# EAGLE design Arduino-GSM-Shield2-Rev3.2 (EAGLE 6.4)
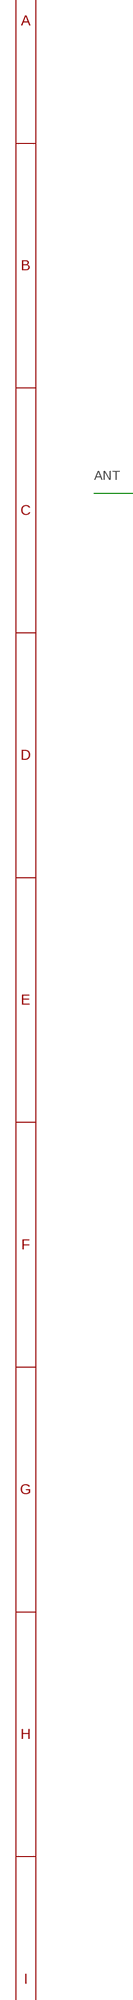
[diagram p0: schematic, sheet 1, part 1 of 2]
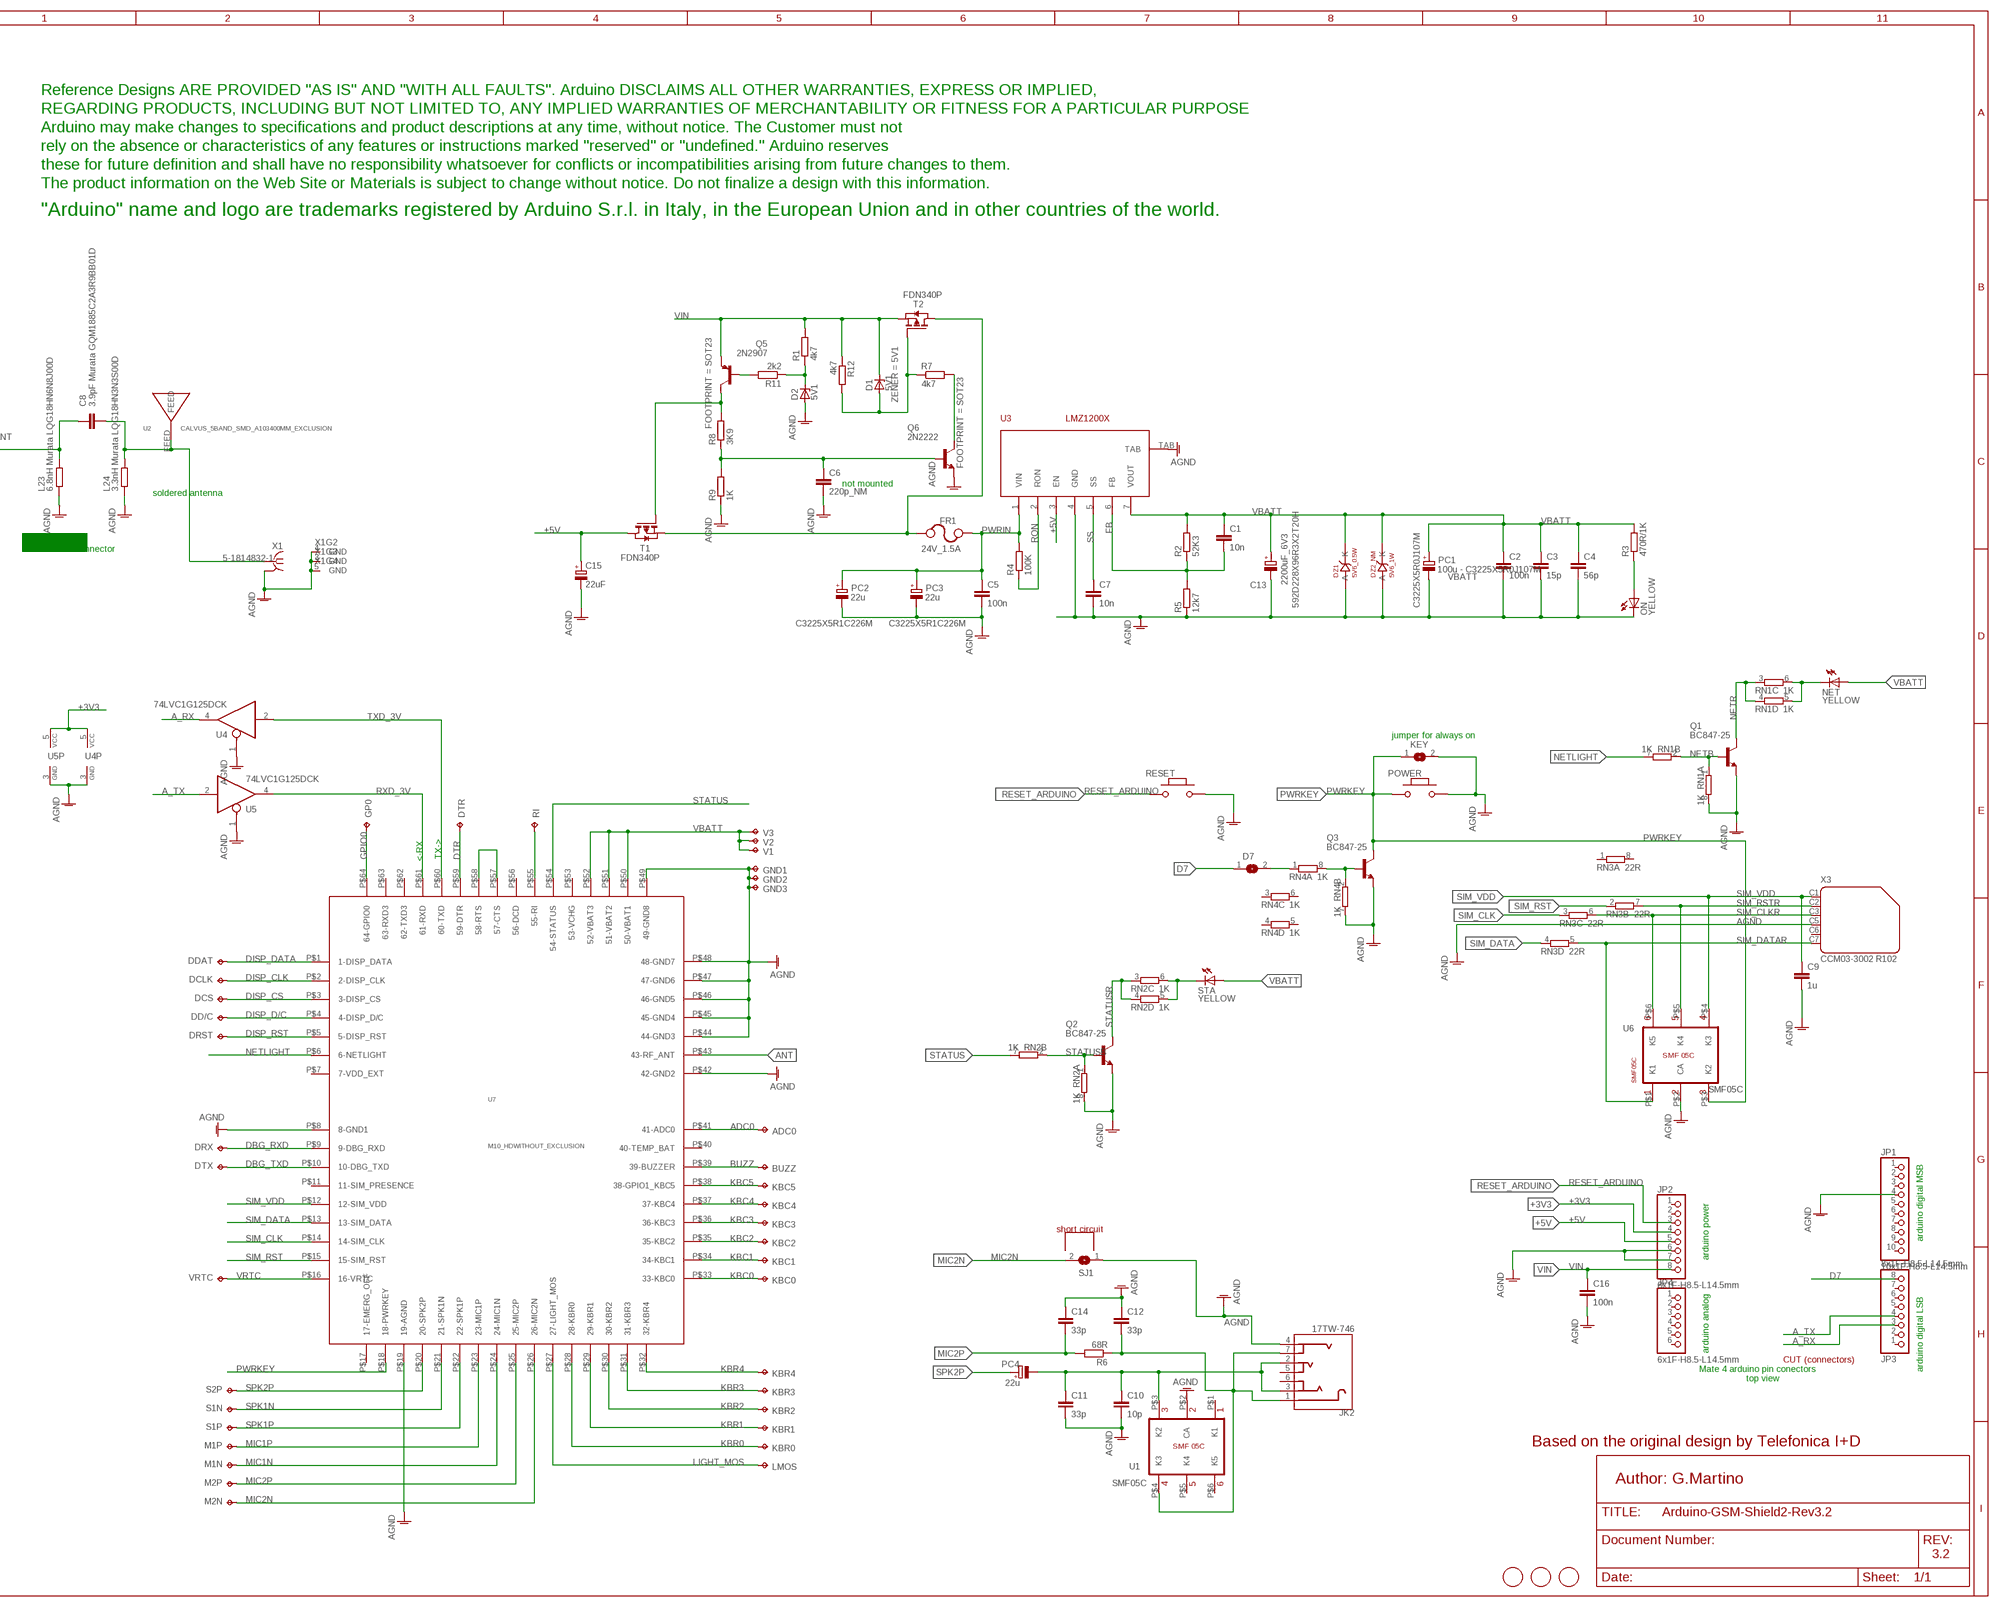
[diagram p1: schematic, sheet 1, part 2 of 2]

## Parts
ADC0  TPPAD1-09  [P1-09]
BUZZ  TPPAD1-09  [P1-09]
C1  10n  C-EU0603-RND  [C0603-ROUND]
C2  100n  C-EU0603-RND  [C0603-ROUND]
C3  15p  C-EU0603-RND  [C0603-ROUND]
C4  56p  C-EU0603-RND  [C0603-ROUND]
C5  100n  C-EU0603-RND  [C0603-ROUND]
C6  220p_NM  C-EU0603-RND  [C0603-ROUND]
C7  10n  C-EU0603-RND  [C0603-ROUND]
C8  3.9pF Murata GQM1885C2A3R9BB01D  C-EU0603-RND  [C0603-ROUND]
C9  1u  C-EU0603-RND  [C0603-ROUND]
C10  10p  C-EU0603-RND  [C0603-ROUND]
C11  33p  C-EU0603-RND  [C0603-ROUND]
C12  33p  C-EU0603-RND  [C0603-ROUND]
C13  2200uF_6V3  0348_  [592D-X]
C14  33p  C-EU0603-RND  [C0603-ROUND]
C15  22uF  0167_  [SMC_B]
C16  100n  C-EU0603-RND  [C0603-ROUND]
D1  5V1  ZENER-DIODESMB  [SMB]
D2  5V1  ZENER-DIODESMB  [SMB]
D7  SJ  [SJ]
DCLK  TPPAD1-09  [P1-09]
DCS  TPPAD1-09  [P1-09]
DD/C  TPPAD1-09  [P1-09]
DDAT  TPPAD1-09  [P1-09]
DRST  TPPAD1-09  [P1-09]
DRX  TPPAD1-09  [P1-09]
DTR  TPPAD1-09  [P1-09]
DTX  TPPAD1-09  [P1-09]
DZ1  5V6_0.5W  0433_BZM55B5V6-TR  [MICROMELF-R]
DZ2_NM  5V6_1W  0433_BZM55B5V6-TR_MINIMELF  [MINIMELF]
FR1  24V_1.5A  0319_MF-MSMF150/24X-2_(24V)  [MF-MSMF-S2]
GND1  TPPAD1-09  [P1-09]
GND2  TPPAD1-09  [P1-09]
GND3  TPPAD1-09  [P1-09]
GP0  TPPAD1-09  [P1-09]
JK2  17TW-746  1819_17TW-746  [17TW-746]
JP1  10x1F-H8.5-L14.5mm  PINHD-1X10TH  [1X10-TH]
JP2  8x1F-H8.5-L14.5mm  PINHD-1X8TH  [1X08-TH]
JP3  8x1F-H8.5-L14.5mm  PINHD-1X8TH  [1X08-TH]
JP4  6x1F-H8.5-L14.5mm  PINHD-1X6TH  [1X06-TH]
KBC0  TPPAD1-09  [P1-09]
KBC1  TPPAD1-09  [P1-09]
KBC2  TPPAD1-09  [P1-09]
KBC3  TPPAD1-09  [P1-09]
KBC4  TPPAD1-09  [P1-09]
KBC5  TPPAD1-09  [P1-09]
KBR0  TPPAD1-09  [P1-09]
KBR1  TPPAD1-09  [P1-09]
KBR2  TPPAD1-09  [P1-09]
KBR3  TPPAD1-09  [P1-09]
KBR4  TPPAD1-09  [P1-09]
KEY  SJ  [SJ]
L23  6.8nH Murata LQG18HN6N8J00D  R-EU_0603-RND  [R0603-ROUND]
L24  3.3nH Murata LQG18HN3N3S00D  R-EU_0603-RND  [R0603-ROUND]
LMOS  TPPAD1-09  [P1-09]
M1N  TPPAD1-09  [P1-09]
M1P  TPPAD1-09  [P1-09]
M2N  TPPAD1-09  [P1-09]
M2P  TPPAD1-09  [P1-09]
NET  YELLOW  LEDCHIP-LED0805  [CHIP-LED0805]
ON  YELLOW  LEDCHIP-LED0805  [CHIP-LED0805]
PC1  100u - C3225X5R0J107M  CPOL-EUSMCB  [SMC_B]
PC2  22u  CPOL-EUSMCB  [SMC_B]
PC3  22u  CPOL-EUSMCB  [SMC_B]
PC4  22u  CPOL-EUSMCB  [SMC_B]
POWER  MYSMD_PB157  [SMD_157SW]
Q1  BC847-25  BC817-25SMD  [SOT23-BEC]
Q2  BC847-25  BC817-25SMD  [SOT23-BEC]
Q3  BC847-25  BC817-25SMD  [SOT23-BEC]
Q5  2N2907  MMBT2907ALT1-PNP-SOT23-BEC  [SOT23-BEC]
Q6  2N2222  MMBT2222ALT1-NPN-SOT23-BEC  [SOT23-BEC]
R1  4k7  R-EU_0603-RND  [R0603-ROUND]
R2  52K3  R-EU_0603-RND  [R0603-ROUND]
R3  470R/1K  R-EU_0603-RND  [R0603-ROUND]
R4  100K  R-EU_0603-RND  [R0603-ROUND]
R5  12k7  R-EU_0603-RND  [R0603-ROUND]
R6  68R  R-EU_0603-RND  [R0603-ROUND]
R7  4k7  R-EU_0603-RND  [R0603-ROUND]
R8  3K9  R-EU_0603-RND  [R0603-ROUND]
R9  1K  R-EU_0603-RND  [R0603-ROUND]
R11  2k2  R-EU_0603-RND  [R0603-ROUND]
R12  4k7  R-EU_0603-RND  [R0603-ROUND]
RESET  MYSMD_PB157  [SMD_157SW]
RI  TPPAD1-09  [P1-09]
RN1  1K  4R-NCAY16  [CAY16]
RN2  1K  4R-NCAY16  [CAY16]
RN3  22R  4R-NCAY16  [CAY16]
RN4  1K  4R-NCAY16  [CAY16]
S1N  TPPAD1-09  [P1-09]
S1P  TPPAD1-09  [P1-09]
S2P  TPPAD1-09  [P1-09]
SJ1  SJ  [SJ]
STA  YELLOW  LEDCHIP-LED0805  [CHIP-LED0805]
T1  FDN340P  PMOSSOT23  [SOT-23]
T2  FDN340P  PMOSSOT23  [SOT-23]
U1  SMF05C  [SC70_6L]
U2  CALVUS_5BAND_SMD_A103400MM_EXCLUSION  [CALVUS_5BAND_SMD_A10340_0MM_EXCLUSION]
U3  LMZ1200X  [TZA-7]
U4  74LVC1G125DCK  [SC70-5]
U5  74LVC1G125DCK  [SC70-5]
U6  SMF05C  [SC70_6L]
U7  M10_HDWITHOUT_EXCLUSION  [M10_HD_WITHOUT_EXCLUSION]
U$1  FIDUCIALMOUNT  [FIDUCIA-MOUNT]
U$2  FIDUCIALMOUNT  [FIDUCIA-MOUNT]
U$3  FIDUCIALMOUNT  [FIDUCIA-MOUNT]
U$4  DISCLAIMER  [DISCLAIMER]
V1  TPPAD1-09  [P1-09]
V2  TPPAD1-09  [P1-09]
V3  TPPAD1-09  [P1-09]
VRTC  TPPAD1-09  [P1-09]
X1  0633_5-1814832-1  [BU-SMA-V]
X3  CCM03-3002 R102  0575_CCM03-3002_R102  [CON-AMPHENOL_C707_10M006_512_2]

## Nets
+3V3: JP2.4 U4.5(VCC) U5.5(VCC)
+5V: C15.+ JP2.5 T1.1(D) U3.3(EN)
A_RX: JP3.3 U4.4(O)
A_TX: JP3.4 U5.2(I)
ADC0: ADC0.TP U7.P$41(41-ADC0)
AGND: C2.2 C3.2 C4.2 C5.2 C6.2 C7.2 C9.2 C10.2 C11.2 C12.1 C13.- C14.1 C15.- C16.2 D2.A DZ1.A DZ2_NM.A GND1.TP GND2.TP GND3.TP JK2.4 JP1.4 JP2.6 JP2.7 KEY.2 L23.1 L24.1 ON.C PC1.- PC2.- PC3.- POWER.2 Q1.E Q2.E Q3.E Q6.E R5.1 R9.1 RESET.2 RN1.8 RN2.8 RN4.7 SJ1.1 U1.P$2(CA) U3.4(GND) U3.TAB U4.1(OE) U4.3(GND) U5.1(OE) U5.3(GND) U6.P$2(CA) U7.P$8(8-GND1) U7.P$19(19-AGND) U7.P$42(42-GND2) U7.P$44(44-GND3) U7.P$45(45-GND4) U7.P$46(46-GND5) U7.P$47(47-GND6) U7.P$48(48-GND7) U7.P$49(49-GND8) X1.2(GND) X1.3(GND) X1.4(GND) X1.5(GND) X3.C5
ANT [antenna]: C8.1 L23.2 U7.P$43(43-RF_ANT)
ANTENA [antenna]: C8.2 L24.2 U2.FEED X1.1
BUZZ: BUZZ.TP U7.P$39(39-BUZZER)
D7: D7.1 JP3.8
DBG_RXD: DRX.TP U7.P$9(9-DBG_RXD)
DBG_TXD: DTX.TP U7.P$10(10-DBG_TXD)
DISP_CLK: DCLK.TP U7.P$2(2-DISP_CLK)
DISP_CS: DCS.TP U7.P$3(3-DISP_CS)
DISP_D/C: DD/C.TP U7.P$4(4-DISP_D/C)
DISP_DATA: DDAT.TP U7.P$1(1-DISP_DATA)
DISP_RST: DRST.TP U7.P$5(5-DISP_RST)
DTR: DTR.TP U7.P$59(59-DTR)
FB: C1.2 R2.1 R5.2 U3.6(FB)
GPIO0: GP0.TP U7.P$64(64-GPIO0)
KBC0: KBC0.TP U7.P$33(33-KBC0)
KBC1: KBC1.TP U7.P$34(34-KBC1)
KBC2: KBC2.TP U7.P$35(35-KBC2)
KBC3: KBC3.TP U7.P$36(36-KBC3)
KBC4: KBC4.TP U7.P$37(37-KBC4)
KBC5: KBC5.TP U7.P$38(38-GPIO1_KBC5)
KBR0: KBR0.TP U7.P$28(28-KBR0)
KBR1: KBR1.TP U7.P$29(29-KBR1)
KBR2: KBR2.TP U7.P$30(30-KBR2)
KBR3: KBR3.TP U7.P$31(31-KBR3)
KBR4: KBR4.TP U7.P$32(32-KBR4)
LIGHT_MOS: LMOS.TP U7.P$27(27-LIGHT_MOS)
MIC1N: M1N.TP U7.P$24(24-MIC1N)
MIC1P: M1P.TP U7.P$23(23-MIC1P)
MIC2N: M2N.TP SJ1.2 U7.P$26(26-MIC2N)
MIC2P: C14.2 M2P.TP R6.2 U7.P$25(25-MIC2P)
N$1: U7.P$57(57-CTS) U7.P$58(58-RTS)
N$2: RI.TP U7.P$55(55-RI)
N$3: ON.A R3.1
N$4: Q3.B RN4.2 RN4.8
N$6: C12.2 JK2.1 JK2.7 R6.1 U1.P$4(K3)
N$7: D7.2 RN4.1
N$8: Q6.C R7.2
N$9: Q5.C R8.2 T1.3(G)
N$10: Q5.B R11.2
N$11: C6.1 Q6.B R8.1 R9.2
N$12: C10.1 C11.1 JK2.2 JK2.3 PC4.- U1.P$3(K2)
N$13: D1.A R7.1 R12.2 T2.3(G)
N$14: D2.C R1.1 R11.1
N$15: FR1.P$1 T1.2(S) T2.1(D)
NETB: Q1.B RN1.1 RN1.2
NETL: NET.C RN1.5 RN1.6
NETLIGHT: RN1.7 U7.P$6(6-NETLIGHT)
NETR: Q1.C RN1.3 RN1.4
PWRIN: C5.1 FR1.P$2 PC2.+ PC3.+ R4.2 U3.1(VIN)
PWRKEY: KEY.1 POWER.1 Q3.C U6.P$3(K2) U7.P$18(18-PWRKEY)
RESET_ARDUINO: JP2.3 RESET.1
RON: R4.1 U3.2(RON)
RXD_3V: U5.4(O) U7.P$61(61-RXD)
SIM_CLK: RN3.3 U7.P$14(14-SIM_CLK)
SIM_CLKR: RN3.6 U6.P$6(K5) X3.C3
SIM_DATA: RN3.4 U7.P$13(13-SIM_DATA)
SIM_DATAR: RN3.5 U6.P$1(K1) X3.C7
SIM_RST: RN3.2 U7.P$15(15-SIM_RST)
SIM_RSTR: RN3.7 U6.P$5(K4) X3.C2
SIM_VDD: C9.1 U6.P$4(K3) U7.P$12(12-SIM_VDD) X3.C1
SPK1N: S1N.TP U7.P$21(21-SPK1N)
SPK1P: S1P.TP U7.P$22(22-SPK1P)
SPK2P: PC4.+ S2P.TP U7.P$20(20-SPK2P)
SS: C7.1 U3.5(SS)
STATUS: RN2.7 U7.P$54(54-STATUS)
STATUSB: Q2.B RN2.1 RN2.2
STATUSL: RN2.5 RN2.6 STA.C
STATUSR: Q2.C RN2.3 RN2.4
TXD_3V: U4.2(I) U7.P$60(60-TXD)
VBATT: C1.1 C2.1 C3.1 C4.1 C13.+ DZ1.C(K) DZ2_NM.C(K) NET.A PC1.+ R2.2 R3.2 STA.A U3.7(VOUT) U7.P$50(50-VBAT1) U7.P$51(51-VBAT2) U7.P$52(52-VBAT3) V1.TP V2.TP V3.TP
VIN: C16.1 D1.C JP2.8 Q5.E R1.2 R12.1 T2.2(S)
VRTC: U7.P$16(16-VRTC) VRTC.TP
Unconnected: JK2.5 JK2.6 JP1.1 JP1.2 JP1.3 JP1.5 JP1.6 JP1.7 JP1.8 JP1.9 JP1.10 JP2.1 JP2.2 JP3.1 JP3.2 JP3.5 JP3.6 JP3.7 JP4.1 JP4.2 JP4.3 JP4.4 JP4.5 JP4.6 RN3.1 RN3.8 RN4.3 RN4.4 RN4.5 RN4.6 U1.P$1(K1) U1.P$5(K4) U1.P$6(K5) U7.P$7(7-VDD_EXT) U7.P$11(11-SIM_PRESENCE) U7.P$17(17-EMERG_OFF) U7.P$40(40-TEMP_BAT) U7.P$53(53-VCHG) U7.P$56(56-DCD) U7.P$62(62-TXD3) U7.P$63(63-RXD3) X3.C6

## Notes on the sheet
- not mounted
- soldered antenna
- SMA or U.FL connector
- 592D228X96R3X2T20H
- jumper for always on
- <-RX
- TX->
- SMF05C
- short circuit
- arduino digital MSB
- arduino power
- arduino analog
- CUT (connectors)
- Mate 4 arduino pin conectors | arduino digital LSB
- top view
- Based on the original design by Telefonica I+D
- Author: G.Martino
- 3.2

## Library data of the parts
ADC0 BUZZ DCLK DCS DD/C DDAT DRST DRX DTR DTX GND1-GND3 GP0 KBC0 KBC1-KBC5 KBR0 KBR1-KBR4 LMOS M1N M1P M2N M2P RI S1N S1P S2P V1-V3 VRTC = testpad:TP: Test pad
C1-C12 C14 C16 = SmartPrj:C-EU: CAPACITOR, European symbol
C13 = Condensatori:0348_: 2200uF 16V Elettr. V � Tantalio; MONTHLY_USAGE: 546.27; TYPE: Condensatori
C15 = Condensatori:0167_: 22uF 25V; MONTHLY_USAGE: 319.15; PRICE: �_0.12; SUPPLIER: La_Tecnika_Due_s.r.l.; TYPE: Condensatori
D1 = diode:ZENER-DIODE: Z-Diode; ZENER: 5V1
D2 = diode:ZENER-DIODE: Z-Diode
D7 KEY = jumper:SJ: SMD solder JUMPER
DZ1 = Diodi:0433_BZM55B5V6-TR: Small Signal Zener Diode BZM55B5V6-TR; CASE: MicroMELF/SOD323/SOD110; MONTHLY_USAGE: 0; PART_NUMBER: BZM55B5V6-TR; SUPPLIER: La_Tecnika_Due_s.r.l.; TYPE: Diodi
DZ2_NM = Diodi:0433_BZM55B5V6-TR: Small Signal Zener Diode BZM55B5V6-TR
FR1 = Protezione:0319_MF-MSMF150/24X-2_(24V): MF-MSMF150/24X-2 (24V) -Polyfuse; MONTHLY_USAGE: 0; PART_NUMBER: MF-MSMF150/24X-2_(24V); PRICE: �_0.11; SUPPLIER: La_Tecnika_Due_s.r.l.; TYPE: Protezione
JK2 = Connettori:1819_17TW-746: Audio Jack 3,5mm for mobiles SMD
JP1 = SmartPrj:PINHD-1X10: PIN HEADER
JP2 JP3 = SmartPrj:PINHD-1X8: PIN HEADER
JP4 = SmartPrj:PINHD-1X6: PIN HEADER
L23 L24 R1-R9 R11 R12 = SmartPrj:R-EU_: RESISTOR, European symbol
NET ON STA = led:LED: LED
PC1 = rcl:CPOL-EU: POLARIZED CAPACITOR, European symbol; PN: C3225X5R0J107M
PC2-PC4 = rcl:CPOL-EU: POLARIZED CAPACITOR, European symbol; PN: C3225X5R1C226M
POWER RESET = SmartPrj:MYSMD_PB157
Q1-Q3 = transistor-npn:BC817*: NPN Transistor
Q5 = transistor-neu-to92:*-PNP-: PNP Transistror; FOOTPRINT: SOT23
Q6 = transistor-neu-to92:*-NPN-: NPN Transistror; FOOTPRINT: SOT23
RN1-RN4 = resistor-dil:4R-N: Array Chip Resistor Source: RS Component / Phycomp
SJ1 = SmartPrj:SJ: SMD solder JUMPER
T1 T2 = zetex:PMOSSOT23: MOS FET
U1 U6 = SmartPrj:SMF05C: SMF05C-TVS Diode Array For ESD and Latch-Up Protection
U2 = SmartPrj:CALVUS_5BAND_SMD_A10340
U3 = SmartPrj:LMZ1200X
U4 U5 = 74xx-little-us:74*1G125: Single Bus Buffer Gate with 3-State Output
U7 = GSM:M10_HD
U$1-U$3 = SmartPrj:FIDUCIALMOUNT
U$4 = Misc:DISCLAIMER
X1 = Connettori:0633_5-1814832-1: SMA STRAIGHT PCB SOCKET DIE CAST; MONTHLY_USAGE: _____; PN: 5-1814832-1; PRICE: _____; SUPPLIER: _____; TYPE: Connettori; VALUE: 5-1814832-1
X3 = Connettori:0575_CCM03-3002_R102: CCM03-3002 R102; MONTHLY_USAGE: _____; PART_NUMBER: CCM03-3002_R102; PRICE: _____; SUPPLIER: _____; TYPE: Connettori

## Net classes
1 power: width 0.305 mm, drill 0.406 mm, clearance 0.178 mm
2 gnd: width 0.305 mm, drill 0.406 mm, clearance 0.178 mm
3 power usb: width 0.508 mm, drill 0.406 mm, clearance 0.178 mm
4 antenna: clearance 0.61 mm

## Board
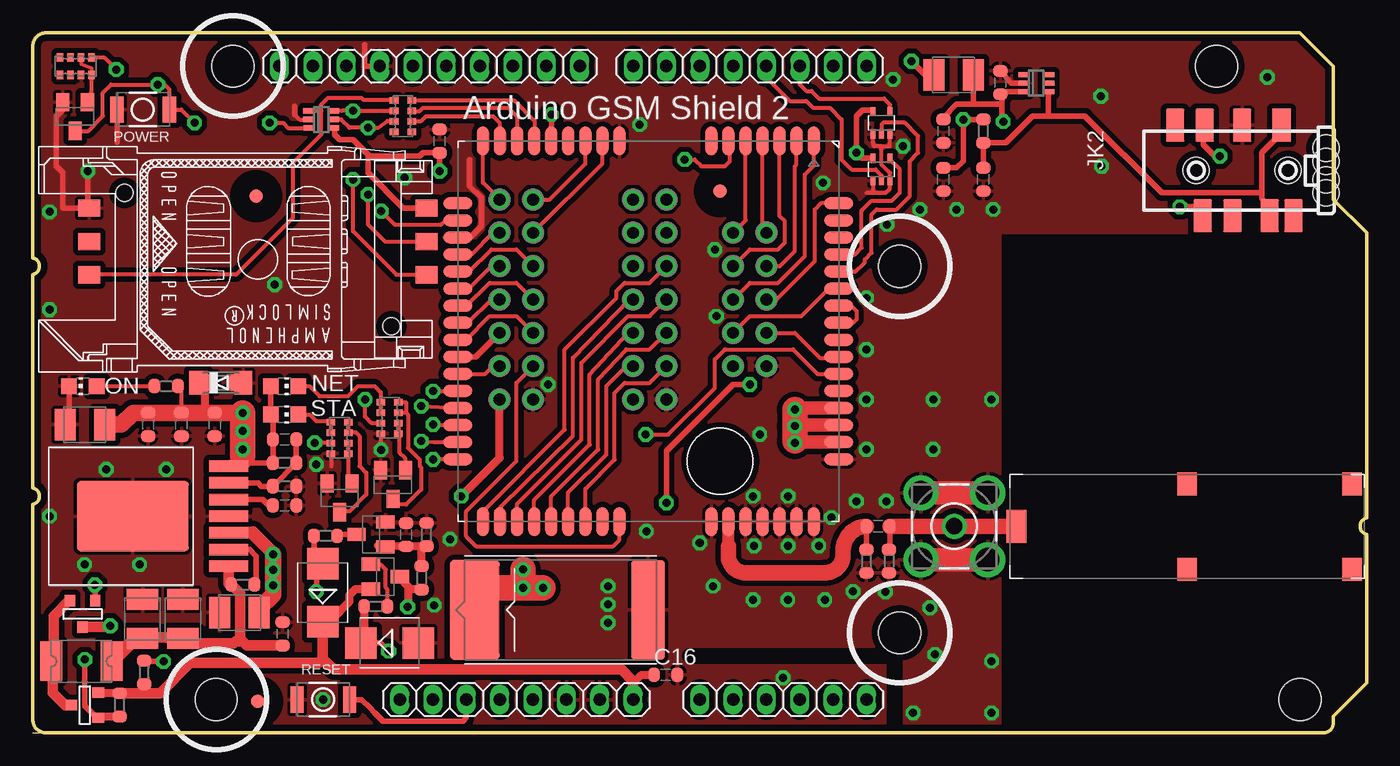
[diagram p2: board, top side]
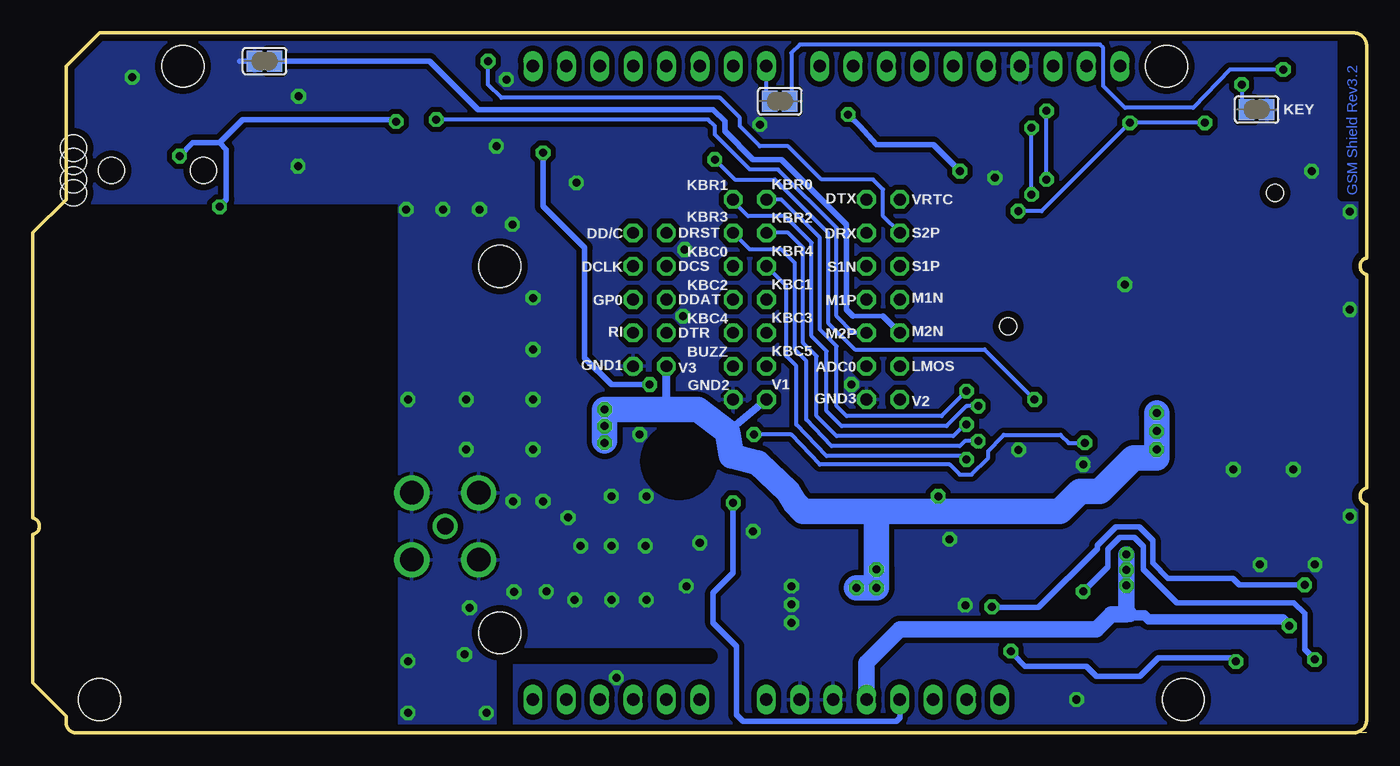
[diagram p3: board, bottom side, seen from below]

Size 101.6 x 53.34 mm. Coordinates in mm from the lower left corner, seen from the top.
Outline: 0,0 77.09,0
Outline: 77.09,0 1,0 arc-90 0,1 0,17.4 arc155 0,18.67 0,34.92 arc155 0,36.2 0,52.34 arc-90 1,53.34 96.52,53.34 99.06,50.8 99.06,40.64 101.6,38.1 101.6,16.38 arc155 101.6,15.11 101.6,3.81 99.06,1.27 99.06,0.76 arc-90 98.3,0 77.09,0
Copper layers (1*16): Top 0.035mm / dielectric 1.5mm / Bottom 0.035mm
Design rules "default *": minimum track width 10mil, minimum drill 24mil, track to track 8mil, track to pad 8mil, pad to pad 8mil, via to via 10mil, smd to smd 8mil, copper to edge 20mil, drill to drill 12mil, minimum pad ring 10mil, minimum via ring 10mil, stop-mask expansion 1mil, vias tented up to drill 30mil, thermal gap 10mil
Holes 3.2 mm at 66.04,35.56 66.04,7.62 15.24,50.8 13.97,2.54 96.52,2.54 90.17,50.8
tRestrict: area 74.9,16.6 to 76.8,18.4; 4 lines
bRestrict: area 0.3,40.9 to 1.8,52.8; 2 lines

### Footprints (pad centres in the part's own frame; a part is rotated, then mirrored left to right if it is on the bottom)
P1-09 = drill 0.9 pad 1.422 octagon: TP 0,0
C0603-ROUND = smd 0.898 x 1.1: 1 -0.889,0; 2 0.889,0
592D-X = smd 7.62 x 3.81: + 0,5.588 | smd 7.62 x 2.54: - 0,-7.62
SMC_B = smd 1.6 x 2.4: + -1.5,0; - 1.5,0
SMB = smd 2.4 x 2.4: A 2.2,0; C -2.2,0
SJ = smd 1.168 x 1.6: 1 -0.762,0; 2 0.762,0
MICROMELF-R = smd 0.8 x 1.2: A 0.8,0; C -0.8,0
MINIMELF = smd 1.4 x 1.8: A 1.7,0; C -1.7,0
MF-MSMF-S2 = smd 1.7 x 3: P$1 -2.3,0; P$2 2.3,0
17TW-746 = smd 1.4 x 2.5: 1 2.8,-3.45; 2 8.8,3.45; 3 8.65,-3.45; 4 5.8,-3.45; 5 10.9,-3.45; 6 6.55,3.45; 7 3.7,3.45; 8 1.9,3.45 | hole 2: 9.3,0; -0.6,1.7; -0.6,-1.7; -0.6,0.7; -0.6,-0.7; 2.3,0
1X10-TH = drill 0.95 pad 1.422 long: 1 -11.43,0; 2 -8.89,0; 3 -6.35,0; 4 -3.81,0; 5 -1.27,0; 6 1.27,0; 7 3.81,0; 8 6.35,0; 9 8.89,0; 10 11.43,0
1X08-TH = drill 0.95 pad 1.422 long: 1 -8.89,0; 2 -6.35,0; 3 -3.81,0; 4 -1.27,0; 5 1.27,0; 6 3.81,0; 7 6.35,0; 8 8.89,0
1X06-TH = drill 0.95 pad 1.422 long: 1 -6.35,0; 2 -3.81,0; 3 -1.27,0; 4 1.27,0; 5 3.81,0; 6 6.35,0
R0603-ROUND = smd 0.898 x 1.1: 1 -0.889,0; 2 0.889,0
CHIP-LED0805 = smd 1.2 x 1.2: A 0,-1.05; C 0,1.05
SMD_157SW = smd 1.016 x 1.981: 1 0,0; 2 4,0
SOT23-BEC = smd 1 x 1.4: B -0.95,-1.1; C 0,1.1; E 0.95,-1.1
CAY16 = smd 0.5 x 0.65: 1 -1.2,-0.675; 2 -0.4,-0.675; 3 0.4,-0.675; 4 1.2,-0.675; 5 1.2,0.675; 6 0.4,0.675; 7 -0.4,0.675; 8 -1.2,0.675
SOT-23 = smd 0.787 x 0.889: 1 0.025,-1.016; 2 -0.94,1.016; 3 0.991,1.016
SC70_6L = smd 0.4 x 0.85: P$1 -0.65,-0.94; P$2 0,-0.94; P$3 0.65,-0.935; P$4 0.65,0.94; P$5 0,0.94; P$6 -0.65,0.94
CALVUS_5BAND_SMD_A10340_0MM_EXCLUSION = smd 2.5 x 1.5: FEED 3.95,0.5 | smd 1.75 x 1.5: FIXINGPOINT$1 0.7,26.05; FIXINGPOINT$2 7.22,26.05; FIXINGPOINT$3 0.7,13.49; FIXINGPOINT$4 7.22,13.49
TZA-7 = smd 0.89 x 3.06: 1 -3.81,-7.305; 2 -2.54,-7.305; 3 -1.27,-7.305; 4 0,-7.305; 5 1.27,-7.305; 6 2.54,-7.305; 7 3.81,-7.305 | smd 5.35 x 8.54: TAB 0,0
SC70-5 = smd 0.4 x 0.7: 1 -0.65,-0.85; 2 0,-0.85; 3 0.65,-0.85; 4 0.65,0.85; 5 -0.65,0.85
M10_HD_WITHOUT_EXCLUSION = smd 2.2 x 0.9: P$1 0,27.1; P$2 0,25.8; P$3 0,24.5; P$4 0,23.2; P$5 0,21.9; P$6 0,20.6; P$7 0,19.3; P$8 0,12.3; P$9 0,11; P$10 0,9.7; P$11 0,8.4; P$12 0,7.1; P$13 0,5.8; P$14 0,4.5; P$15 0,3.2; P$16 0,1.9; P$33 29,1.9; P$34 29,3.2; P$35 29,4.5; P$36 29,5.8; P$37 29,7.1; P$38 29,8.4; P$39 29,9.7; P$40 29,11; P$41 29,12.3; P$42 29,19.3; P$43 29,20.6; P$44 29,21.9; P$45 29,23.2; P$46 29,24.5; P$47 29,25.8; P$48 29,27.1 | smd 0.9 x 2.2: P$17 4.75,0; P$18 6.05,0; P$19 7.35,0; P$20 8.65,0; P$21 9.95,0; P$22 11.25,0; P$23 12.55,0; P$24 13.85,0; P$25 15.15,0; P$26 16.45,0; P$27 17.75,0; P$28 19.05,0; P$29 20.35,0; P$30 21.65,0; P$31 22.95,0; P$32 24.25,0; P$49 24.25,29; P$50 22.95,29; P$51 21.65,29; P$52 20.35,29; P$53 19.05,29; P$54 17.75,29; P$55 16.45,29; P$56 15.15,29; P$57 13.85,29; P$58 12.55,29; P$59 11.25,29; P$60 9.95,29; P$61 8.65,29; P$62 7.35,29; P$63 6.05,29; P$64 4.75,29
FIDUCIA-MOUNT = smd 1.016 x 1.016: P$1 0,0
BU-SMA-V = drill 1.27: 1 0,0 | drill 1.778: 2 -2.55,2.55; 3 2.55,2.55; 4 2.55,-2.55; 5 -2.55,-2.55
CON-AMPHENOL_C707_10M006_512_2 = smd 1.7 x 1.3: C1 -12.85,-3.915; C2 -12.85,-1.375; C3 -12.85,1.165; C5 12.85,-3.915; C6 12.85,-1.375; C7 12.85,1.165 | hole 1.3: 10.16,-5.08; -10.16,5.08

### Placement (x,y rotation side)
ADC0  38.1,27.94 0 top
BUZZ  48.26,27.94 0 top
C1  19.18,22.35 0 top
C2  8.78,23.5 270 top
C3  13.86,23.5 270 top
C4  11.32,23.5 270 top
C5  19.02,7.54 90 top
C6  28.44,15.1 90 top
C7  19.18,17.32 0 top
C8  64.39,15.75 0 top
C9  30.99,45.09 90 top
C10  73.71,49.56 90 top
C11  69.34,45.85 270 top
C12  72.39,42.16 90 top
C13  39.24,9.37 90 top
C14  69.34,42.16 90 top
C15  15.75,9.17 180 top
C16  48.21,4.42 0 top
D1  22.09,10.69 90 top
D2  27.18,6.85 0 top
D7  44.7,48.13 0 bottom
DCLK  55.88,35.56 0 top
DCS  53.34,35.56 0 top
DD/C  55.88,38.1 0 top
DDAT  53.34,33.02 0 top
DRST  53.34,38.1 0 top
DRX  38.1,38.1 0 top
DTR  53.34,30.48 0 top
DTX  38.1,40.64 0 top
DZ1  14.35,26.7 0 top
DZ2_NM  14.33,26.67 0 top
FR1  3.71,5.46 0 top
GND1  55.88,27.94 0 top
GND2  48.26,25.4 0 top
GND3  38.1,25.4 0 top
GP0  55.88,33.02 0 top
JK2  97.92,42.85 180 top
JP1  30.23,50.8 0 top
JP2  36.83,2.54 0 top
JP3  54.61,50.8 180 top
JP4  57.15,2.54 0 top
KBC0  48.26,35.56 0 top
KBC1  45.72,33.02 0 top
KBC2  48.26,33.02 0 top
KBC3  45.72,30.48 0 top
KBC4  48.26,30.48 0 top
KBC5  45.72,27.94 0 top
KBR0  45.72,40.64 0 top
KBR1  48.26,40.64 0 top
KBR2  45.72,38.1 0 top
KBR3  48.26,38.1 0 top
KBR4  45.72,35.56 0 top
KEY  8.38,47.5 0 bottom
L23  63.5,13.08 90 top
L24  65.23,13.08 90 top
LMOS  35.56,27.94 0 top
M1N  35.56,33.02 0 top
M1P  38.1,33.02 0 top
M2N  35.56,30.48 0 top
M2P  38.1,30.48 0 top
NET  19.18,26.42 270 top
ON  3.81,26.42 90 top
PC1  3.97,23.5 180 top
PC2  8.36,8.69 90 top
PC3  11.43,8.69 90 top
PC4  70.13,50.14 0 top
POWER  10.41,47.5 180 top
Q1  27.43,18.92 180 top
Q2  23.37,17.91 180 top
Q3  3.22,46.96 180 top
Q5  26.86,11.9 270 top
Q6  25.77,15.12 90 top
R1  8.48,4.61 270 top
R2  19.18,20.57 180 top
R3  10.16,26.42 0 top
R4  16,11.3 180 top
R5  19.18,18.8 180 top
R6  72.39,45.85 90 top
R7  22.29,15.02 0 top
R8  29.63,11.81 270 top
R9  29.99,15.11 270 top
R11  26.12,9.64 0 top
R12  6.61,2.13 270 top
RESET  24.13,2.54 180 top
RI  55.88,30.48 0 top
RN1  27.18,24 90 top
RN2  23.37,22.48 90 top
RN3  28.19,46.99 90 top
RN4  3.27,50.8 180 top
S1N  38.1,35.56 0 top
S1P  35.56,35.56 0 top
S2P  35.56,38.1 0 top
SJ1  83.95,51.18 0 bottom
STA  19.18,24.26 270 top
T1  3.76,9.07 0 top
T2  3.96,2.14 270 top
U1  76.43,49.5 270 top
U2  74.42,19.68 270 top
U3  7.62,16.51 90 top
U4  64.64,46.48 0 top
U5  64.64,42.93 0 top
U6  21.97,46.74 270 top
U7  32.38,45.1 270 top
U$1  17.02,40.89 0 top
U$2  52.32,41.27 0 top
U$3  17.11,2.4 0 top
U$4  not placed on the board
V1  45.72,25.4 0 top
V2  35.56,25.4 0 top
V3  53.34,27.94 0 top
VRTC  35.56,40.64 0 top
X1  70.18,15.75 0 top
X3  17.14,36.07 180 top

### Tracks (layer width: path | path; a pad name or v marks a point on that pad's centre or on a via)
+3V3  (via drill 0.61)
  Top 0.305: 63.99,47.43 U4.5
  Top 0.406: v48.26,17.53 48.26,21.46 53.34,26.54 v54.61,26.54 | U5.5 63.16,43.78 v62.74,44.2 62.74,46.99 63.18,47.43 63.99,47.43
  Bottom 0.406: v62.74,44.2 62.74,40.13 59.56,36.96 59.56,28.57 57.53,26.54 v54.61,26.54 | v48.26,17.53 48.26,12.19 49.78,10.67 49.78,8.38 48.01,6.6 48.01,1.4 47.5,0.89 35.81,0.89 35.56,1.14 JP2.4
+5V  (via drill 0.61)
  Top 0.813: 5.87,8.1 v5.89,8.15 5.87,8.05 5.33,8.08 3.81,8.08 T1.1
  Top 0.914: 16.76,15.24 U3.3
  Top 1.016: 16.76,15.24 18.16,13.84 v18.29,13.61
  Top 1.27: v18.29,13.61 v18.29,12.42 v18.29,11.23 | v18.29,11.23 18.29,11.18 | C15.+ 17.25,9.48 18.29,10.52 v18.29,11.23
  Bottom 0.406: 18.01,8.99 18.16,9.14
  Bottom 0.813: 17.98,8.97 16.94,8.97 16.61,8.64 6.38,8.64 v5.89,8.15
  Bottom 1.016: 18.01,8.99 17.98,8.97
  Bottom 1.27: v18.29,13.61 v18.29,11.23 18.29,9.02 | 18.16,9.14 18.29,9.02 | JP2.5 38.1,5.33 35.56,7.87 20.57,7.87 19.43,9.02 18.29,9.02
A_RX
  Top 0.305: U4.4 65.29,47.86 64.83,48.32 59.88,48.32 59.31,48.9 58.93,48.9 58.42,49.4 JP3.3
A_TX
  Top 0.305: U5.2 64.64,42.47 64.19,42.93 62.36,42.93 61.59,43.69 61.59,46.74 60.71,47.62 59.44,47.62 58.93,48.13 57.66,48.13 55.88,49.91 JP3.4
ADC0
  Top 0.305: U7.P$41 44.69,14.71 44.2,14.22 33.78,14.22 33.02,14.99 33.02,16.89 36.83,20.7 36.83,26.67 ADC0.TP
AGND  (via drill 0.61, 0.61 pad 0.81)
  Top 0.305: 64.64,44.7 65.28,44.7 65.28,45.62 U4.3 | U5.1 63.99,41.16 63.5,41.15 64.96,41.15 65.28,41.47 65.28,42.06 U5.3 65.29,42.66 64.64,43.31 64.64,44.7 | 64.64,44.7 64.07,44.7 64.01,45.02 64.01,45.62 U4.1 | Q3.E 2.46,48.56 | RN4.7 3.68,50.11 | RN2.8 arc90 22.73,21.19 22.73,20.32 | U6.P$2 20.32,46.74 19.94,47.12 | 26.63,21.42 v26.52,21.57 26.5,21.63 RN1.8
  Top 0.406: U7.P$19 33.3,37.75 34.16,38.61 34.16,40.77 33.27,41.66 33.27,43.69 | 6.41,45.02 POWER.2 | v4.19,42.8 4.19,40.09 X3.C5 2.27,39.98 2.29,42.67 1.78,43.18 1.78,46.99 2.27,47.48 Q3.E | ON.C 2.76,23.84 PC1.- | JP1.4 25.27,50.8 25.27,52.45 | 19.94,47.12 19.94,47.75 | U1.P$2 74.55,49.51 C10.2
  Top 0.813: C15.- 13.87,9.02
  Top 1.778: X1.5 X1.4 | X1.2 X1.3
  Bottom 0.406: SJ1.1 85.83,51.18
  other vias: 54.94,14.25 57.53,14.25 60.83,16.41 59.87,14.25 54.86,10.13 57.51,10.13 60.33,10.13 62.48,10.77 50.8,14.48 51.82,11.18 62.74,17.65 73.03,5.46 68.33,9.53 64.95,10.74 67.06,1.52 73.03,1.52 68.58,21.59 43.81,9.78 60.2,41.91 63.5,21.59 63.5,25.4 63.5,29.21 63.5,33.15 65.07,38.73 67.56,39.88 1.27,39.7 1.27,32.26 1.27,16.51 31.78,14.76 46.74,15.37 54.86,18.03 57.53,18.03 55.37,22.73 57.15,4.19 10.16,20.07 5.59,20.07 3.94,12.83 8.13,12.83 18.41,34.16 46.23,46.35 39.24,26.54 52.07,31.75 28.32,42.29 65.02,17.65 68.58,25.4 73.03,25.4 68.71,5.97 51.94,36.83 65.53,49.78 81.36,48.51 66.29,44.7 70.36,39.88 73.15,39.88 81.41,43.18 30.58,9.73 43.81,11.18 43.81,8.38 22.1,2.54 21.59,20.45 94.03,49.96
  pour Bottom (isolate 0.406): -0.51,54.86 100.2,54.86 100.2,40.39 73.66,40.39 73.66,-0.38 -0.25,-0.25 -0.51,-0.25
  pour Top (isolate 0.406): -0.51,54.86 99.57,54.99 99.57,38.13 73.66,38.13 73.66,-0.38 -0.51,-0.38
ANT
  Top 0.406: C8.1 L23.2
  Top 0.914: 52.98,14.22 U7.P$43
  Top 1.168: 52.98,14.22 52.98,13.72 arc90 54.13,12.19 60.33,12.19 arc90 61.72,13.59 61.72,13.84 arc-90 C8.1
ANTENA
  Top 0.406: 65.53,15.53 C8.2 65.28,13.97 L24.2
  Top 1.168: U2.FEED arc90 74.78,15.75 X1.1 C8.2
BUZZ
  Top 0.305: U7.P$39 42.09,18.59 44.32,20.83 44.32,25.91 45.09,26.67 46.99,26.67 BUZZ.TP
D7
  Bottom 0.305: D7.1 45.72,48.13 45.72,48.77 JP3.8
DBG_RXD
  Top 0.305: U7.P$9 43.38,43.38 DRX.TP
DBG_TXD
  Top 0.305: U7.P$10 42.09,43.35 39.37,40.64 DTX.TP
DISP_CLK
  Top 0.305: DCLK.TP 56.9,35.56 58.04,36.7 58.04,43.18 58.17,43.31 58.17,45.08 U7.P$2
DISP_CS
  Top 0.305: U7.P$3 56.88,39.38 57.28,38.99 57.28,37.34 56.77,36.83 54.61,36.83 DCS.TP
DISP_D/C
  Top 0.305: U7.P$4 55.59,38.4 DD/C.TP
DISP_DATA
  Top 0.305: U7.P$1 59.48,43.23 58.8,42.55 58.8,36.32 56.77,34.29 54.61,34.29 DDAT.TP
DISP_RST
  Top 0.305: U7.P$5 54.28,39.05 DRST.TP
DTR
  Top 0.305: U7.P$59 60.65,33.85 58.55,31.75 54.61,31.75 DTR.TP
FB
  Top 0.406: U3.6 17.14,19.05 17.4,18.8 R5.2 R2.1 C1.2
GPIO0
  Top 0.305: GP0.TP 56.64,33.02 59.56,35.94 59.56,39.88 60.07,40.39 61.35,40.39 U7.P$64
KBC0
  Top 0.305: U7.P$33 34.28,16.89 40.51,23.11 40.51,29.21 44.45,33.15 44.45,33.66 45.09,34.29 46.99,34.29 KBC0.TP
KBC1
  Top 0.305: U7.P$34 35.59,17.17 41.15,22.61 41.15,28.57 45.47,33.02 KBC1.TP
KBC2
  Top 0.305: U7.P$35 36.88,17.45 41.78,22.35 41.78,28.19 45.34,31.75 46.99,31.75 KBC2.TP
KBC3
  Top 0.305: U7.P$36 38.19,17.74 42.42,21.97 42.42,27.3 45.34,30.48 KBC3.TP
KBC4
  Top 0.305: U7.P$37 39.48,18.02 43.05,21.59 43.05,26.92 45.21,29.21 46.99,29.21 KBC4.TP
KBC5
  Top 0.305: U7.P$38 40.78,18.31 43.69,21.21 43.69,26.42 45.21,27.94 KBC5.TP
KBR0  (via drill 0.61)
  Top 0.305: U7.P$28 32.37,26.04 v30.48,26.04
  Bottom 0.305: v30.48,26.04 32.38,24.13 39.62,24.13 40.39,24.89 40.39,29.46 41.66,30.73 41.66,37.72 44.58,40.64 KBR0.TP
KBR1  (via drill 0.61)
  Top 0.305: U7.P$29 32.37,24.77 v29.59,24.89
  Bottom 0.305: v29.59,24.89 30.48,24.89 32,23.37 40.01,23.37 41.15,24.51 41.15,29.08 42.29,30.23 42.29,37.34 44.32,39.37 47.12,39.37 48.26,40.51 KBR1.TP
KBR2  (via drill 0.61)
  Top 0.305: U7.P$30 30.52,23.45 v30.48,23.5
  Bottom 0.305: KBR2.TP 44.07,38.1 42.93,36.96 42.93,29.72 41.91,28.7 41.91,24.13 40.39,22.61 31.5,22.61 30.61,23.5 v30.48,23.5
KBR3  (via drill 0.61)
  Top 0.305: U7.P$31 30.55,22.15 v29.59,22.23
  Bottom 0.305: KBR3.TP 46.99,36.83 44.58,36.83 43.56,35.81 43.56,29.21 42.67,28.32 42.67,23.88 40.77,21.84 30.99,21.84 30.61,22.23 v29.59,22.23
KBR4  (via drill 0.61)
  Top 0.305: U7.P$32 30.63,20.85 v30.48,20.83
  Bottom 0.305: KBR4.TP 44.2,34.04 44.2,28.7 43.43,27.94 43.43,23.5 41.15,21.08 30.73,21.08 v30.48,20.83 30.63,20.85
LIGHT_MOS
  Top 0.305: U7.P$27 34.46,27.35 35.05,27.94 LMOS.TP
MIC1N
  Top 0.305: U7.P$24 33.16,31.25 34.92,33.02 M1N.TP
MIC1P
  Top 0.305: M1P.TP 36.83,34.29 34.8,34.29 33.06,32.55 U7.P$23
MIC2N
  Top 0.406: U7.P$26 33.73,28.65 M2N.TP
  Bottom 0.356: 36.83,31.75 39.12,31.75
  Bottom 0.406: M2N.TP 36.83,31.75 | 39.12,31.75 39.62,32.26 39.62,38.73 44.58,43.69 46.74,43.69 48.9,45.85 48.9,46.61 49.78,47.5 67.69,47.5 71.37,51.18 SJ1.2
  Bottom 0.61: SJ1.2 84.33,51.18
MIC2P  (via drill 0.61)
  Top 0.305: M2P.TP 36.83,31.75 34.8,31.75 33,29.95 U7.P$25
  Top 0.406: C14.2 70.36,43.05 70.87,43.56 v70.87,46.74 R6.2
  Bottom 0.305: M2P.TP 39.12,30.48 40.39,31.75 40.39,38.48 44.83,42.93 46.99,42.93 49.66,45.59 49.66,46.23 50.16,46.74 v70.87,46.74
N$1
  Top 0.305: U7.P$58 62.32,32.55 62.74,32.13 62.74,31.5 62.48,31.24 61.39,31.24 U7.P$57
N$2
  Top 0.305: RI.TP 58.04,30.48 59.94,28.57 61.31,28.57 U7.P$55
N$3
  Top 0.305: ON.A R3.1
N$4
  Top 0.254: RN4.2 3.67,50.94 4.47,50.65 RN4.8
  Top 0.305: RN4.8 4.47,48.87 Q3.B
N$6
  Top 0.406: C12.2 R6.1 74.12,44.96 76.15,46.99 77.47,46.99 | 93.6,41.15 93.6,44.2 94.61,45.21 94.61,45.34 95,45.72 95,46.18 JK2.1 | 93.6,41.15 93.6,40.78 JK2.7 | 77.47,46.99 80.14,46.99 85.98,41.15 93.6,41.15 | U1.P$4 77.37,47.09 77.47,46.99
N$7  (via drill 0.61)
  Top 0.305: RN4.1 5.42,51.48 v6.35,50.55
  Bottom 0.305: D7.2 43.81,48.51 43.81,51.82 43.18,52.45 20.32,52.45 20.07,52.2 20.07,49.28 18.41,47.62 13.21,47.62 10.41,50.55 v6.35,50.55
N$8
  Top 0.406: Q6.C 23.28,15.12 R7.2
N$9  (via drill 0.61)
  Top 0.406: v4.72,11.28 4.75,11.2 T1.3
  Top 0.61: 28.4,9.75 v28.55,9.6 28.6,9.65 28.6,10.92 | Q5.C 27.96,11.77 28.6,11.12 28.6,10.92 | R8.2 28.6,10.92
  Bottom 0.406: v28.55,9.6 28.5,9.55 24.99,9.55 20.52,14.02 20.52,14.28 19.1,15.7 17.32,15.7 16.31,14.68 16.31,12.95 15.14,11.79 10.21,11.79 9.7,11.28 v4.72,11.28
N$10
  Top 0.305: R11.2 27.01,10.93 26.87,11.07 26.87,12.45 26.52,12.8 25.81,12.8 Q5.B
N$11
  Top 0.305: 27.92,14.06 C6.1
  Top 0.61: R8.1 29.63,14.06 R9.2 27.92,14.22 C6.1 26.29,14.26 Q6.B
N$12  (via drill 0.61)
  Top 0.406: 73.77,46.52 v73.91,46.58 73.81,46.69 73.81,47.9 | C10.1 74.2,48.85 U1.P$3 | 73.77,48.42 C10.1 | C11.1 69.34,46.89 70.36,47.9 71.73,47.9 | 71.73,47.9 73.81,47.9 | PC4.- 71.63,48.01 71.73,47.9 | C10.1 73.81,48.56 73.81,47.9 | v87.38,40.08 88.98,40.08 89.15,40.13 89.03,40.33 JK2.2 | JK2.3 89.15,47.17 89.15,44.83 90.04,43.94 v90.42,43.94
  Bottom 0.406: v73.91,46.58 74.12,46.58 74.27,46.74 85.6,46.74 87.38,44.96 | v87.38,40.08 87.25,40.26 86.87,40.64 86.87,44.45 87.38,44.96 | 87.38,44.96 89.41,44.96 v90.42,43.94
N$13  (via drill 0.61)
  Top 0.406: R7.1 21.45,13.73 D1.A 21.64,12.48 v21.59,10.77 | 5.2,1.2 T2.3 | 5.07,1.24 4.81,1.24 3.96,2.08 v3.96,5.59
  Top 0.61: 21.78,13.48 21.95,13.31 21.95,13.24 D1.A | R12.2 5.07,1.24 T2.3
  Bottom 0.406: v21.59,10.77 19.71,12.65 19.71,13.97 18.8,14.88 17.68,14.88 17.02,14.22 17.02,12.45 14.48,9.91 5.54,9.91 4.72,9.09 4.72,6.35 v3.96,5.59
N$14  (via drill 0.61)
  Top 0.406: D2.C 26.48,6.85 v27.1,6.22 | R1.1 8.55,5.44 v9.96,5.44
  Top 0.61: R11.1 25.24,7.2 D2.C
  Bottom 0.406: v27.1,6.22 26.92,5.97 26.04,5.08 21.34,5.08 20.57,4.32 17.27,4.32 15.88,5.71 10.36,5.71 10.03,5.44 v9.96,5.44
N$15
  Top 0.813: T1.2 2.77,10.08 1.57,8.89 1.57,5.53 FR1.P$1 1.52,5.45 1.52,3.05 2.46,2.11 T2.1
NETB
  Top 0.305: Q1.B 28.38,20.89 27.94,21.34 27.94,22.72 RN1.1 RN1.2
NETL
  Top 0.305: NET.C 21.08,26.42 21.84,25.65 24,25.65 24.77,26.42 26.04,26.42 26.5,25.95 RN1.5 RN1.6
NETLIGHT  (via drill 0.61)
  Top 0.305: v49.66,43.69 50.42,43.69 50.93,43.18 52.7,43.18 53.09,43.56 53.09,44.32 52.96,44.45 52.96,45.07 U7.P$6 | v25.3,25.4 25.3,24.11 25.78,23.62 26.48,23.62 RN1.7
  Bottom 0.305: v49.66,43.69 48.13,42.16 45.09,42.16 41.02,38.1 41.02,31.24 38.99,29.21 29.11,29.21 v25.3,25.4
NETR
  Top 0.305: 28.45,24.38 28.57,24.26 28.57,21.72 29.46,20.83 29.46,20.32 29.59,20.19 29.59,18.54 28.45,17.4 27.39,17.4 Q1.C | 28.45,24.38 27.87,24.38 RN1.3 | RN1.4 28.39,25.2 28.45,25.15 28.45,24.38
PWRIN
  Top 0.813: U3.1 14.93,11.49 | 14.93,11.49 R4.2 15.8,10.62 15.8,6.96 | 14.93,11.49 14.93,11.36 | 15.8,6.96 15.44,6.96 15.29,6.81 11.68,6.81 11.23,7.26 8.76,7.26 PC3.+ | 15.8,6.96 16,6.96 16.31,6.66 C5.1
  Top 1.016: 8.33,7.11 PC2.+ | PC2.+ 8.53,7.03 8.76,7.26 | FR1.P$2 7.84,7.19 PC2.+
PWRKEY  (via drill 0.61)
  Top 0.305: U7.P$18 31.43,39.05 31.11,38.73 27.56,38.73 v26.54,39.75 | Q3.C 4.2,45.86 5.33,46.99 5.33,48.77 5.97,49.4 v9.53,49.4 10.03,49.4 10.41,49.02 POWER.1 11.3,47.5 v12.32,46.48 | U6.P$3 19.45,46.09 19.05,46.48 v18.03,46.48
  Bottom 0.305: v26.54,39.75 24.77,39.75 v18.03,46.48 v12.32,46.48 | v9.53,49.4 9.53,47.88 KEY.1
RESET_ARDUINO
  Top 0.406: RESET.1 25.04,2.54 25.68,1.91 26.04,1.52 26.67,0.89 32.77,0.89 33.02,1.14 JP2.3
RON
  Top 0.406: U3.2 16.51,13.97 17.02,13.46 17.02,11.18 R4.1
RXD_3V
  Top 0.305: U7.P$61 62.61,36.45 63.12,36.96 63.12,39.77 63.88,40.54 65.43,40.54 66.04,41.15 66.04,42.95 65.34,43.65 U5.4
SIM_CLK
  Top 0.305: U7.P$14 36.88,46.94 36.2,47.62 29.72,47.62 29.46,47.37 28.89,47.37 RN3.3
SIM_CLKR  (via drill 0.61)
  Top 0.305: X3.C3 27.71,34.9 24.38,38.23 v24.38,42.16 | U6.P$6 23.55,47.39 v24.38,47.39 RN3.6
  Bottom 0.305: v24.38,42.16 v24.38,47.39
SIM_DATA
  Top 0.305: U7.P$13 38.23,45.14 38.23,46.61 36.65,48.19 RN3.4
SIM_DATAR
  Top 0.305: X3.C7 15.47,34.9 19.81,39.24 19.81,43.43 21.97,45.59 21.97,47.39 | 21.97,47.39 21.97,47.88 22.48,48.39 25.02,48.39 25.15,48.26 27.45,48.26 RN3.5 | 21.97,47.39 U6.P$1
SIM_RST
  Top 0.305: RN3.2 29.59,46.61 29.95,46.97 35.07,46.97 35.56,46.48 35.56,45.12 U7.P$15
SIM_RSTR  (via drill 0.61)
  Top 0.305: X3.C2 26.82,37.44 25.53,38.73 v25.53,41.02 | U6.P$5 23.5,46.74 24.13,46.1 v25.53,46.1 26.29,46.1 26.99,46.61 27.5,46.61 RN3.7
  Bottom 0.305: v25.53,41.02 v25.53,46.1
SIM_VDD  (via drill 0.61)
  Top 0.406: 25.53,44.07 25.65,43.94 29.46,43.94 29.72,44.2 C9.1 v30.99,42.8 | U7.P$12 39.48,45.33 v39.5,47.12 | X3.C1 28.22,39.98 25.53,42.67 25.53,44.07 | U6.P$4 22.99,46.01 22.99,45.59 23.37,45.21 24.38,45.21 25.53,44.07
  Bottom 0.406: v30.99,42.8 33.02,44.83 37.34,44.83 38.61,46.23 v39.5,47.12
SPK1N
  Top 0.305: S1N.TP 36.83,36.83 34.92,36.83 33.24,35.15 U7.P$21
SPK1P
  Top 0.305: U7.P$22 33.22,33.85 34.92,35.56 S1P.TP
SPK2P  (via drill 0.61)
  Top 0.305: U7.P$20 33.4,36.45 35.05,38.1 S2P.TP
  Top 0.406: PC4.+ 68.48,49.63 v66.93,51.18
  Bottom 0.305: S2P.TP 36.83,39.37 36.83,41.4 37.59,42.16 41.53,42.16 44.07,44.7 46.23,44.7 47.75,46.23 47.75,46.86 49.28,48.39 65.91,48.39 66.93,49.4 v66.93,51.18
SS
  Top 0.406: U3.5 17.5,17.78 18.06,17.22 C7.1
STATUS  (via drill 0.61)
  Top 0.305: U7.P$54 59.77,27.35 57.91,29.21 52.7,29.21 51.94,28.45 51.94,26.29 48.39,22.73 v46.69,22.73 | RN2.7 22.71,22.08 22.73,22.1 v21.46,22.1
  Bottom 0.305: v46.69,22.73 43.81,22.73 41.66,20.45 31.75,20.45 30.99,19.68 30.1,19.68 28.83,20.95 28.83,21.46 27.76,22.58 27.64,22.71 23.32,22.71 RN2.7 21.48,22.08 v21.46,22.1
STATUSB
  Top 0.305: RN2.2 RN2.1 24.04,18.65 Q2.B
  Top 0.406: Q2.B 24.42,18.5
STATUSL
  Top 0.305: RN2.6 RN2.5 22.75,23.75 21.59,23.75 21.08,24.26 STA.C
STATUSR
  Top 0.305: RN2.4 RN2.3 24.62,22.88 24.89,22.61 24.89,20.32 25.4,19.81 25.4,18.16 24.13,16.89 23.45,16.89 Q2.C 23.28,16.26
TXD_3V
  Top 0.305: U4.2 64.64,46.35 64.77,46.48 66.42,46.48 67.44,45.47 67.44,44.2 66.8,43.56 66.8,40.89 65.79,39.88 64.26,39.88 63.88,39.5 63.88,36.58 63.37,36.07 63.37,35.85 62.67,35.15 U7.P$60
VBATT  (via drill 0.61)
  Top 0.305: C4.1 11.32,26.4 R3.2
  Top 0.406: NET.A STA.A 18.29,23.97 C1.1 R2.2 16.26,20.57 16,20.45 | DZ2_NM.C 12.95,26.67 13.08,26.54
  Top 0.61: V2.TP 35.56,20.95 v32.64,18.03 | DZ1.C 13.08,26.54 13.08,24.38
  Top 0.813: C13.+ 33.66,10.54 34.16,11.05
  Top 0.914: U3.7 16,20.32 16,20.45
  Top 1.016: 16,21.08 16,20.45 | U7.P$50 58.24,22.15 58.04,22.23 | U7.P$51 58.08,23.45 v58.04,23.37 | U7.P$52 58.05,24.75 v58.04,24.64
  Top 1.27: v16,24.38 C3.1 13.08,24.38 C4.1 C2.1 7.63,24.38 6.74,23.5 PC1.+
  Top 1.93: v16,22.99 16,21.08 | v16,22.99 16,24.26 | v58.04,24.64 v58.04,23.37 58.04,22.23 | v16,24.38 v16,22.99 | v37.34,11.05 v38.86,11.05 | v37.34,11.05 v37.34,12.45 | v37.34,11.05 34.16,11.05
  Bottom 0.61: 53.34,24.64 V3.TP | 32.64,16.89 v32.64,18.03 | 58.04,22.23 v58.04,22.1 | 48.7,22.92 V1.TP
  Bottom 1.676: 37.34,16.76 37.21,16.89
  Bottom 1.93: v16,24.38 v16,21.59 16,20.95 17.78,20.95 20.32,18.41 21.84,18.41 23.37,16.89 32.64,16.89 37.21,16.89 42.93,16.89 43.56,17.53 44.07,18.41 46.35,20.57 48.39,21.08 48.7,22.92 50.93,24.64 53.34,24.64 v58.04,24.64 58.04,22.23 | v38.86,11.05 v37.34,11.05 v37.34,12.45 37.34,16.76
VIN
  Top 0.61: D1.C 22.75,8.04 22.75,8.63 24.13,10.01 24.13,10.52 24.59,10.97 25.74,10.97 Q5.E | 45.72,3.94 45.8,3.94 46.33,4.42 C16.1 | 5.12,3.13 T2.2 5.04,3.02 R12.1
  Top 0.813: 22.3,7.75 D1.C 22.09,5.65 | JP2.8 45.72,3.94 44.83,4.83 22.96,4.83 22.91,4.88 22.09,5.65 | 8.48,3.02 9.45,3.02 9.69,3.03 11.99,5.33 21.78,5.33 22.09,5.65 | 8.48,3.02 R12.1 | R1.2 8.48,3.02
VRTC
  Top 0.305: U7.P$16 34.28,41.91 VRTC.TP

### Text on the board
Bottom: GSM Shield Rev3.2
tPlace: Arduino GSM Shield 2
